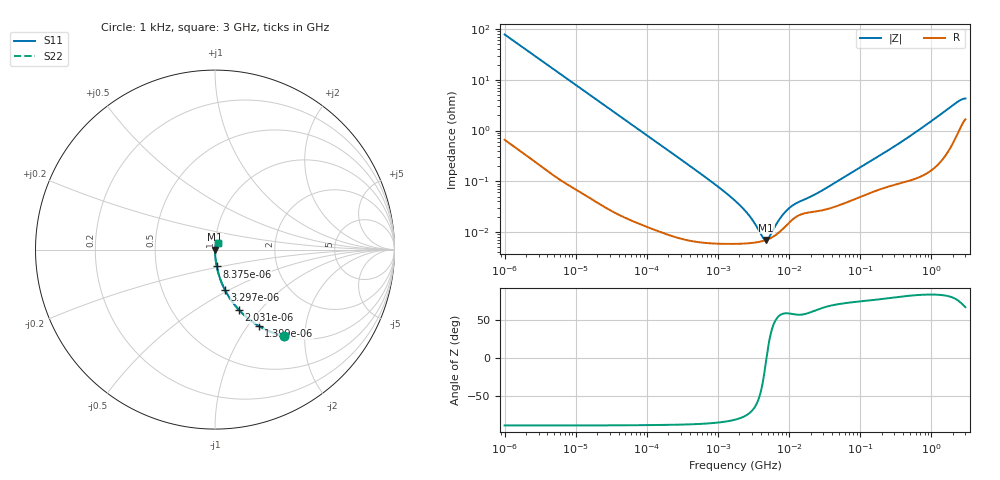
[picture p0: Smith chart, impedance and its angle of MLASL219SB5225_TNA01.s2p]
! MLASL219SB5225_TNA01  S-PARAMETER MODEL  ( Standard Model )
! Model Generated by TAIYO YUDEN Corporation (http://www.ty-top.com)
! Version 1.0
! TAIYO YUDEN Control No. 220601
! Copyright(c) 2009 TAIYO YUDEN CO.,LTD. All Rights Reserved.
! Product Description (link to TY-COMPAS)
! https://ds.yuden.co.jp/TYCOMPAS/or/detail?pn=MLASL219SB5225KTNA01&u=M
! Products Name : Multilayer Ceramic Capacitors
! Characteristics :
!  Capacitance : 2.2 [uF] , Rated Voltage : 10 [V] , TCC : X5R
!  Case Size : 2.0 x 1.25 / 0.079 x 0.049 [mm/inch] , Thickness : 0.85 / 0.033 [mm/inch]
!  (Conditions: Temperature = 25 [degC] , DC Bias Voltage = 0 [V])
! External Node Assignments :
!  1  o---| |---o  2
! GND o---------o GND
! Frequency Range : 1kHz  -  3GHz  [ 401 STEP ]
# MHZ S RI R 50
! Freq[MHz].  S11 Real  S11 Imag  S21 Real  S21 Imag  S12 Real  S12 Imag  S22 Real  S22 Imag
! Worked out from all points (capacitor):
!   401 points, 1 kHz to 3 GHz, reference 50 ohm
!   read as one part in series: C = 2.02 uF near 1.077 kHz
!   lowest |Z| = 6.94 mohm at 4.74 MHz (marker M1)
!   series resonance near 4.806 MHz, so ESL is about 540 pH
!   S11 on the Smith chart (normalised r, x): 1 kHz: 1.01, -1.57; 1.399 kHz: 1.01, -1.13; 2.031 kHz: 1.01, -0.78; 3.297 kHz: 1.00, -0.48; 8.375 kHz: 1.00, -0.19; 3 GHz: 1.03, +0.08
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0.001  0.383 -0.4819  0.617 0.4819  0.617 0.4819  0.383 -0.4819
0.001399  0.2426 -0.4245  0.7574 0.4245  0.7574 0.4245  0.2426 -0.4245
0.002031  0.1333 -0.3358  0.8667 0.3358  0.8667 0.3358  0.1333 -0.3358
0.003297  0.0561 -0.2261  0.9439 0.2261  0.9439 0.2261  0.0561 -0.2261
0.008375  0.0097 -0.0939  0.9903 0.0939  0.9903 0.0939  0.0097 -0.0939
0.01216  0.00484 -0.0651  0.9952 0.0651  0.9952 0.0651  0.00484 -0.0651
0.147855  0.000132 -0.00545  0.9999 0.00545  0.9999 0.00545  0.000132 -0.00545
0.762639  6.08e-05 -0.00104  0.9999 0.00104  0.9999 0.00104  6.08e-05 -0.00104
1.732051  5.83e-05 -0.00041  0.9999 0.00041  0.9999 0.00041  5.83e-05 -0.00041
2.610246  5.96e-05 -0.000221  0.9999 0.000221  0.9999 0.000221  5.96e-05 -0.000221
3.789741  6.36e-05 -8.23e-05  0.9999 8.23e-05  0.9999 8.23e-05  6.36e-05 -8.23e-05
4.083148  6.51e-05 -5.63e-05  0.9999 5.63e-05  0.9999 5.63e-05  6.51e-05 -5.63e-05
4.739869  6.93e-05 -4.74e-06  0.9999 4.74e-06  0.9999 4.74e-06  6.93e-05 -4.74e-06
5.711239  7.78e-05 6e-05  0.9999 -6e-05  0.9999 -6e-05  7.78e-05 6e-05
7.988506  0.000112 0.000179  0.9999 -0.000179  0.9999 -0.000179  0.000112 0.000179
10.37087  0.00016 0.000263  0.9998 -0.000263  0.9998 -0.000263  0.00016 0.000263
12.97096  0.000204 0.000317  0.9998 -0.000317  0.9998 -0.000317  0.000204 0.000317
21.06097  0.000247 0.00045  0.9998 -0.00045  0.9998 -0.00045  0.000247 0.00045
256.0921  0.00081 0.00413  0.9992 -0.00413  0.9992 -0.00413  0.00081 0.00413
675.1638  0.00131 0.0103  0.9987 -0.0103  0.9987 -0.0103  0.00131 0.0103
2226.275  0.00866 0.0339  0.9913 -0.0339  0.9913 -0.0339  0.00866 0.0339
3000  0.0179 0.0382  0.9821 -0.0382  0.9821 -0.0382  0.0179 0.0382
